PROGRAM MAIN
VAR
	PMC01 : PMControllerType;	
	PMC01IN AT %IB0 : ARRAY[0..399] OF BYTE;
	PMC01OUT AT %QB0 : ARRAY[0..399] OF BYTE;	
	PMC_AutoRefresh_DB : PMC_AutoRefresh;	
	
	//Change this to match the actual location of the demo files on your machine
	DemoFilesFolder : STRING := 'C:\Users\TestPlatform\Desktop\TC_Lib_Dev\Demo Files';
	
	FileExample01 : FileExample01_Gcode; FileExample01_run : BOOL; FileExample01_done : BOOL;
	FileExample02 : FileExample02_readlogs; FileExample02_run : BOOL; FileExample02_done : BOOL;
	FileExample03 : FileExample03_Trajectory; FileExample03_run : BOOL; FileExample03_done : BOOL;
	FileExample04 : FileExample04_Configuration; FileExample04_run : BOOL; FileExample04_done : BOOL;
END_VAR

//Initialize with location of fieldbus in and out
PMC01.DataFromPMC := ADR(PMC01IN);
PMC01.DataToPMC := ADR(PMC01OUT);
//maintains fieldbus data for PMCLIB to function properly, only needs to by called once per cycle
PMC_AutoRefresh_DB(Enable := TRUE,PM_Controller := PMC01);

//Examples (comment out examples that are not in use to reduce processor load)
FileExample01(Execute := FileExample01_run,DemoFilesFolder := 'C:\Users\TestPlatform\Desktop\TC_Lib_Dev\Demo Files',Done => FileExample01_done,PM_Controller := PMC01);
//FileExample02(Execute := FileExample02_run,DemoFilesFolder := 'C:\Users\TestPlatform\Desktop\TC_Lib_Dev\Demo Files',Done => FileExample02_done,PM_Controller := PMC01);
//FileExample03(Execute := FileExample03_run,DemoFilesFolder := 'C:\Users\TestPlatform\Desktop\TC_Lib_Dev\Demo Files',Done => FileExample03_done,PM_Controller := PMC01);
//FileExample04(Execute := FileExample04_run,DemoFilesFolder := 'C:\Users\TestPlatform\Desktop\TC_Lib_Dev\Demo Files',Done => FileExample04_done,PM_Controller := PMC01);

END_PROGRAM
